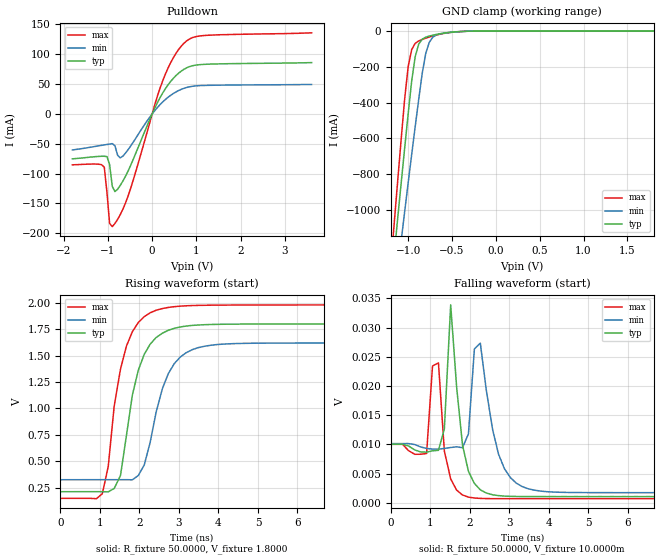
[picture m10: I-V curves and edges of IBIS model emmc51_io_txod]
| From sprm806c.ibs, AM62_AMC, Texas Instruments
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|   Model emmc51_io_txod
[Model]  emmc51_io_txod
Model_type I/O_open_drain
Polarity   Non-Inverting
Enable   Active-High
Vinl =   0.6300V
Vinh =   1.1700V
Vmeas =  0.2000V
Cref =   0.5000pF
Rref =   50.0000
Vref =   0.2000V
C_comp   2.0000pF   2.0000pF   2.0000pF
[Temperature Range]   25.0000   0.1250k   -40.0000
[Voltage Range]   1.8000V   1.6200V   1.9800V
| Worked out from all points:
|   slope of the pulldown table from 0 to 0.27 V, typ, clamps not added: 6.94 ohm
|   GND clamp passes 1 mA (typ) near -0.33 V on its own axis
|   rising waveform, R_fixture 50.0000, V_fixture 1.8000: 20-80 % time 506ps typ, 575ps min, 469ps max; typ from 0.212 V to 1.8 V
[Pulldown]
|Voltage   I(typ)   I(min)   I(max)
-1.8V     -75.19mA   -60.29mA   -85.22mA
-1.08V    -70.83mA   -51.82mA   -89.4mA
-960mV    -84.87mA   -50.43mA   -183.4mA
-900mV    -121.3mA   -49.66mA   -188.7mA
-840mV    -130mA     -53.18mA   -183.5mA
-780mV    -126.1mA   -69.04mA   -176.7mA
-660mV    -112.3mA   -70.56mA   -159.5mA
240mV     35.36mA    20.23mA    55.8mA
480mV     59.86mA    34.36mA    94.5mA
720mV     74.95mA    43.04mA    118.6mA
1.2V      83.23mA    47.87mA    131.6mA
3.6V      86.08mA    49.46mA    136mA
[GND_clamp]
|Voltage   I(typ)   I(min)   I(max)
-1.8V     -4.6A      -4.237A    -5.082A
-1.16V    -1.252A    -1.504A    -1.079A
-1.12V    -1.05A     -1.338A    -840.1mA
-1.08V    -850.3mA   -1.173A    -605.5mA
-1.04V    -654mA     -1.01A     -379.4mA
-1V       -462.2mA   -848.6mA   -198.6mA
-920mV    -143mA     -534.3mA   -68.61mA
-880mV    -73.46mA   -382.5mA   -55.43mA
-800mV    -34.42mA   -125.7mA   -40.22mA
-760mV    -28.09mA   -63.79mA   -33.86mA
-640mV    -15.4mA    -16.09mA   -18.11mA
1.8V      142.8nA    88.96uA    15.91nA
[Ramp]
| variable   typ   min   max
dV/dt_r  0.9531/0.5056n   0.7769/0.5652n   1.0991/0.4593n
dV/dt_f  0.9531/0.2737n   0.7769/0.4329n   1.0991/0.1885n
R_load = 50.0000
[Rising Waveform]
R_fixture= 50.0000
V_fixture= 1.8000
V_fixture_min= 1.6200
V_fixture_max= 1.9800
|time   V(typ)   V(min)   V(max)
0s        211.5mV    325mV      148.2mV
1.06ns    211.7mV    325.3mV    192.7mV
1.21ns    210.2mV    325.2mV    450.6mV
1.36ns    242.1mV    325.2mV    1.021V
1.52ns    364.5mV    325.2mV    1.373V
1.97ns    1.361V     364.5mV    1.813V
2.42ns    1.671V     962.4mV    1.929V
2.88ns    1.758V     1.423V     1.964V
3.79ns    1.794V     1.597V     1.977V
15ns      1.8V       1.62V      1.98V
[Falling Waveform]
R_fixture= 50.0000
V_fixture= 10.0000m
V_fixture_min= 10.0000m
V_fixture_max= 10.0000m
|time   V(typ)   V(min)   V(max)
0s        10.01mV    10.13mV    10mV
910ps     8.655mV    9.299mV    8.425mV
1.21ns    8.972mV    9.175mV    23.96mV
1.36ns    12.65mV    9.295mV    8.841mV
1.52ns    33.89mV    9.454mV    4.077mV
1.82ns    9.848mV    9.416mV    1.316mV
2.12ns    3.302mV    26.34mV    793.5uV
2.42ns    1.659mV    19.36mV    702.2uV
3.64ns    1.045mV    2.144mV    682.9uV
15ns      1.04mV     1.718mV    683.1uV
